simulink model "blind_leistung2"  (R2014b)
settings: Solver=ode8  StartTime=0.0  StopTime=5  FixedStep=1e-5  RelTol=1e-3
undefined symbols (not defined in the file or in its folder): dfilt, fdesignblkfcn, gcbh
libraries: dsparch4 x3

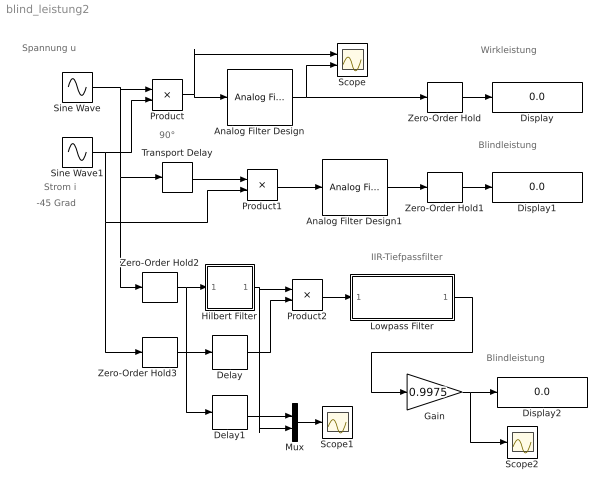
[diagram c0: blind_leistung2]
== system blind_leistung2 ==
  note: IIR-Tiefpassfilter
  note: Blindleistung
  note: Blindleistung
  note: Wirkleistung
  note: 90°
  note: -45 Grad
  note: Strom i
  note: Spannung u
  Analog Filter Design : dsparch4/Analog Filter Design  method=Butterworth  filttype=Lowpass  N=8  Wlo=2*pi*10  Whi=80  Rp=2  Rs=80
  Analog Filter Design1 : dsparch4/Analog Filter Design  method=Butterworth  filttype=Lowpass  N=8  Wlo=2*pi*10  Whi=80  Rp=2  Rs=40
  Delay : Delay  DelayLength=32
  Delay1 : Delay  DelayLength=32
  Display : Display
  Display1 : Display
  Display2 : Display
  Gain : Gain  Gain=0.9975
  Hilbert Filter : Subsystem  DialogController=fdesignblkfcn  InitFcn=fdesignblkfcn(gcbh, {'InitFcn'});
  Lowpass Filter : Subsystem  DialogController=fdesignblkfcn  InitFcn=fdesignblkfcn(gcbh, {'InitFcn'});
  Mux : Mux  Inputs=2
  Product : Product
  Product1 : Product
  Product2 : Product
  Scope : Scope  NumInputPorts=2
  Scope1 : Scope
  Scope2 : Scope
  Sine Wave : Sin  Amplitude=220  Frequency=2*pi*50  SampleTime=0
  Sine Wave1 : Sin  Amplitude=10.52  Frequency=2*pi*50  Phase=-45*pi/180  SampleTime=0
  Transport Delay : TransportDelay  DelayTime=1/200
  Zero-Order Hold{,1..3} (4 alike) : ZeroOrderHold  SampleTime=1/1000
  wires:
  Sine Wave/1 -> Zero-Order Hold2/1, Transport Delay/1, Product/1
  Sine Wave1/1 -> Zero-Order Hold3/1, Product1/2, Product/2
  Product/1 -> Scope/1, Analog Filter Design/1
  Analog Filter Design/1 -> Scope/2, Zero-Order Hold/1
  Zero-Order Hold/1 -> Display/1
  Transport Delay/1 -> Product1/1
  Product1/1 -> Analog Filter Design1/1
  Zero-Order Hold1/1 -> Display1/1
  Analog Filter Design1/1 -> Zero-Order Hold1/1
  Zero-Order Hold2/1 -> Delay1/1, Hilbert Filter/1(In)
  Zero-Order Hold3/1 -> Delay/1
  Hilbert Filter/1(Out) -> Mux/2, Product2/1
  Delay/1 -> Product2/2
  Gain/1 -> Scope2/1, Display2/1
  Mux/1 -> Scope1/1
  Delay1/1 -> Mux/1
  Product2/1 -> Lowpass Filter/1(In)
  Lowpass Filter/1(Out) -> Gain/1

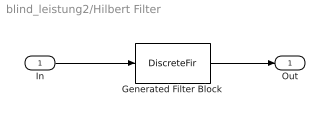
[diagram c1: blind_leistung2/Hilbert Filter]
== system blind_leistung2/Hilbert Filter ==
  In : Inport
  Generated Filter Block : DiscreteFir  Tag=BlockMethodSubSystem  Coefficients=[9.88658825704986609e-06 -0.002227584536743819 -2.97041880887335789e-07 -0.00253443852532551223 3.1215106945712904e-06 -0.00391748816900691285 3.49128676163899538e-06 -0.00575534109882602785 4.57452034469855664e-06 -0.00814133649362377108 5.16425058718461533e-06 -0.0111912068195077624 4.30131386161312988e-06 -0.0150623213220996768 4.89965903312141859e-06 -0.0199570171297331345 4.81145735332042261e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
  Out : Outport
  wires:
  Generated Filter Block/1 -> Out/1
  In/1 -> Generated Filter Block/1

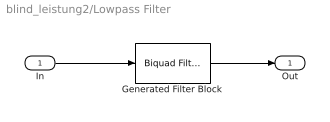
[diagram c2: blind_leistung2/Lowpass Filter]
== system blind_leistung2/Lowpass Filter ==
  In : Inport
  Generated Filter Block : dsparch4/Biquad Filter  Tag=BlockMethodSubSystem  IIRFiltStruct=Direct form II  CoeffSource=Specify via dialog  BiQuadCoeffs=[0.001228643771917717 0.001228643771917717 0 1 -0.981968654161641474 0;0.000658678061035388764 0.00131735612207077753 0.000658678061035388764 1 -1.98494966484313462 0.988828349815104368;0.250214146609910537 0.500428293219821074 0.250214146609910537 1 -1.96932783564244662 0.97099845116727479]  a0Flag=Warning  IC=0  ICnum=0  ICden=0  InputProcessing=Columns as channels (frame based)  denAccumFracLength=30  denProdOutputFracLength=30  secondMemoryFracLength=15  roundingMode=Floor  overflowMode=off  ScaleValues=[0.0180313458383585257;1;1;1]  optimizeScaleValues=off  ScaleValueMode=Specify via input port (g)  scaleValueFracLength=14  FilterSource=Specify via dialog  dfiltObjectName=dfilt.df2tsos([1 0.3 0.4],[1 0.1 0.2])
  Out : Outport
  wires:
  In/1 -> Generated Filter Block/1
  Generated Filter Block/1 -> Out/1
